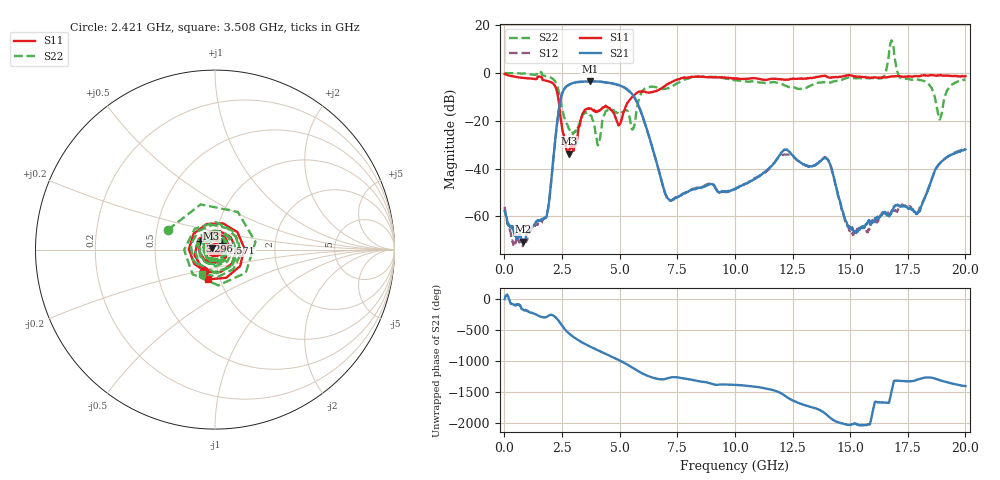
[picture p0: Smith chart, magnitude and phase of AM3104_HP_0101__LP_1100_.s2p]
!Created with skrf (http://scikit-rf.org).
# Hz S RI R 50.0
!freq ReS11 ImS11 ReS21 ImS21 ReS12 ImS12 ReS22 ImS22
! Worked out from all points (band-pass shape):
!   1601 points, 10 MHz to 20 GHz, reference 50 ohm
!   highest |S21| = -3.46 dB at 3.708 GHz (marker M1); lowest = -70.6 dB at 822.1 MHz (marker M2)
!   |S21| within 3 dB of the highest: 2.613 GHz to 5.267 GHz (2.653 GHz wide, 67.3 % of centre)
!   lowest |S11| = -33.7 dB at 2.796 GHz (marker M3), VSWR 1.04, Z = 48.1 + j0.665 ohm
!   |S11| at or under -10 dB: 2.329 GHz to 5.56 GHz (3.231 GHz wide, 81.9 % of centre)
!   |S22| runs from -30.3 to 13.6 dB; largest |S21 - S12| = 0.058
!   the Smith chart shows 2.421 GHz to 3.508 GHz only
!   S11 on the Smith chart (normalised r, x): 2.421 GHz: 0.86, -0.21; 2.571 GHz: 1.08, +0.08; 3.296 GHz: 0.84, +0.08; 3.508 GHz: 0.88, -0.30
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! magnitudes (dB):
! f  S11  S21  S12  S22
! 10 MHz  -0.4  -57.7  -56.0  -0.1
! 822.1 MHz  -2.0  -70.6  -70.1  -0.2
! 1.847 GHz  -3.3  -59.4  -58.7  -1.3
! 2.421 GHz  -17.4  -11.8  -11.9  -10.9
! 2.571 GHz  -25.8  -7.1  -7.1  -17.6
! 2.796 GHz  -33.7  -4.9  -4.9  -23.3
! 3.296 GHz  -20.2  -3.7  -3.8  -19.9
! 3.346 GHz  -18.6  -3.6  -3.7  -18.5
! 3.508 GHz  -15.4  -3.6  -3.6  -16.3
! 3.708 GHz  -14.9  -3.5  -3.5  -17.6
! 5.545 GHz  -10.2  -8.9  -8.9  -23.7
! 6.682 GHz  -7.2  -40.1  -40.1  -6.2
! 7.169 GHz  -4.2  -53.2  -53.4  -6.1
! 10.01 GHz  -2.4  -48.6  -48.7  -3.1
! 12.17 GHz  -2.8  -32.1  -34.1  -5.2
! 13.34 GHz  -2.1  -39.1  -39.1  -5.0
! 14.03 GHz  -1.7  -36.2  -36.2  -4.0
! 15.05 GHz  -1.0  -65.0  -65.8  -1.9
! 16.68 GHz  -1.6  -59.8  -58.9  7.3
! 17.95 GHz  -1.3  -58.2  -58.1  -2.7
! 18.89 GHz  -1.0  -37.9  -37.9  -19.4
! 20 GHz  -1.3  -32.0  -31.4  -2.8
